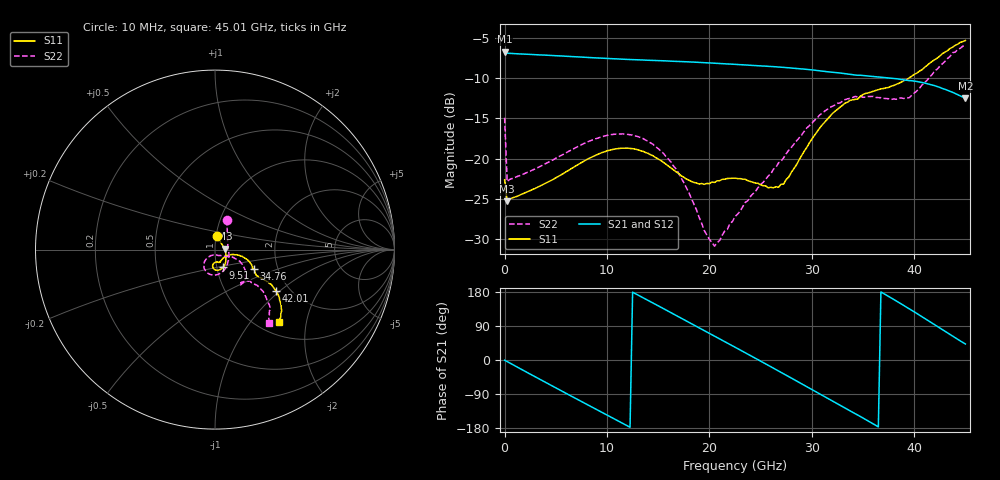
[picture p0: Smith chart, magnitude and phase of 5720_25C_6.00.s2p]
! Device:  ADRF5720
! Description: 0.5dB LSB GaAs MMIC 6-bit Digital Attenuator
! Frequency:  0.000009 -  40 GHz
! Ports:
!	RF1	= Port 1
!	RF2	= Port 2
! Vdd:  3.3 Volt
! Vss:  -3.3 Volt
! Control:  0/3.3 Volt
! State:  6.00 dB attenuation
! Data:  The device was measured using G-S-G Probes on a matrix board.
!  Data was collected using an calibrated 4 port network analyzer.
!  The reference plane for this measurement is at the launchers.
! Note:  Analog Devices supplies this data as a sample of measured data
!  for this product.  Your particular data for this product may vary.
!  Data was taken at 25 degrees C.
!  Analog Devices reserves the right to change this data at anytime.
# GHZ S DB R 45.0
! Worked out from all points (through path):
!   181 points, 10 MHz to 45.01 GHz, reference 45 ohm
!   highest |S21| = -6.75 dB at 10 MHz (marker M1); lowest = -12.5 dB at 45.01 GHz (marker M2)
!   group delay of S21, straight-line fit = 41.3 ps
!   lowest |S11| = -25.3 dB at 260 MHz (marker M3), VSWR 1.12, Z = 50.2 + j0.559 ohm
!   |S11| at or under -10 dB: start of sweep to 39.51 GHz
!   |S22| runs from -30.8 to -5.9 dB; largest |S21 - S12| = 0.00052
!   S11 on the Smith chart (normalised r, x): 10 MHz: 1.01, +0.15; 9.51 GHz: 1.07, -0.22; 34.76 GHz: 1.51, -0.35; 42.01 GHz: 1.70, -0.94; 45.01 GHz: 1.23, -1.40
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0.01  -22.62 82.1  -6.75 -0.6  -6.75 -0.6  -14.93 68.6
0.26  -25.26 5.8  -6.94 -4.1  -6.94 -4.1  -22.84 3.3
2.26  -24.09 -15.5  -7.07 -33.6  -7.08 -33.6  -21.68 -19.4
4.26  -22.89 -31.1  -7.20 -62.6  -7.20 -62.6  -20.46 -37.9
6.01  -21.62 -42.5  -7.31 -87.9  -7.31 -87.9  -19.27 -52.0
7.76  -20.30 -53.7  -7.43 -113.1  -7.43 -113.1  -18.12 -65.6
9.51  -19.25 -65.6  -7.55 -138.1  -7.55 -138.1  -17.29 -79.4
12.51  -18.76 -85.8  -7.73 179.0  -7.73 179.0  -17.08 -103.6
15.26  -20.22 -97.5  -7.86 139.4  -7.87 139.4  -19.04 -123.8
18.01  -22.66 -92.8  -8.02 99.6  -8.02 99.6  -24.24 -133.4
19.51  -23.18 -82.7  -8.11 77.7  -8.11 77.7  -28.90 -118.2
20.51  -22.95 -76.9  -8.18 63.1  -8.18 63.1  -30.84 -89.2
22.76  -22.47 -70.4  -8.34 30.2  -8.34 30.2  -26.88 -46.7
24.76  -23.05 -61.9  -8.49 0.8  -8.49 0.8  -23.59 -34.5
26.76  -23.54 -39.2  -8.65 -28.9  -8.65 -28.9  -20.52 -25.1
30.26  -17.14 -13.3  -9.04 -81.5  -9.05 -81.5  -15.27 -28.3
32.51  -13.89 -19.3  -9.35 -115.4  -9.35 -115.4  -13.15 -38.6
34.76  -12.27 -26.4  -9.67 -149.2  -9.67 -149.2  -12.28 -50.1
37.76  -11.02 -32.1  -10.03 163.9  -10.04 164.0  -12.68 -52.8
39.51  -10.00 -31.3  -10.33 135.5  -10.33 135.6  -12.47 -47.5
42.01  -7.75 -34.2  -10.96 92.9  -10.95 92.9  -9.16 -40.9
45.01  -5.36 -48.6  -12.52 42.2  -12.52 42.3  -5.90 -53.6
